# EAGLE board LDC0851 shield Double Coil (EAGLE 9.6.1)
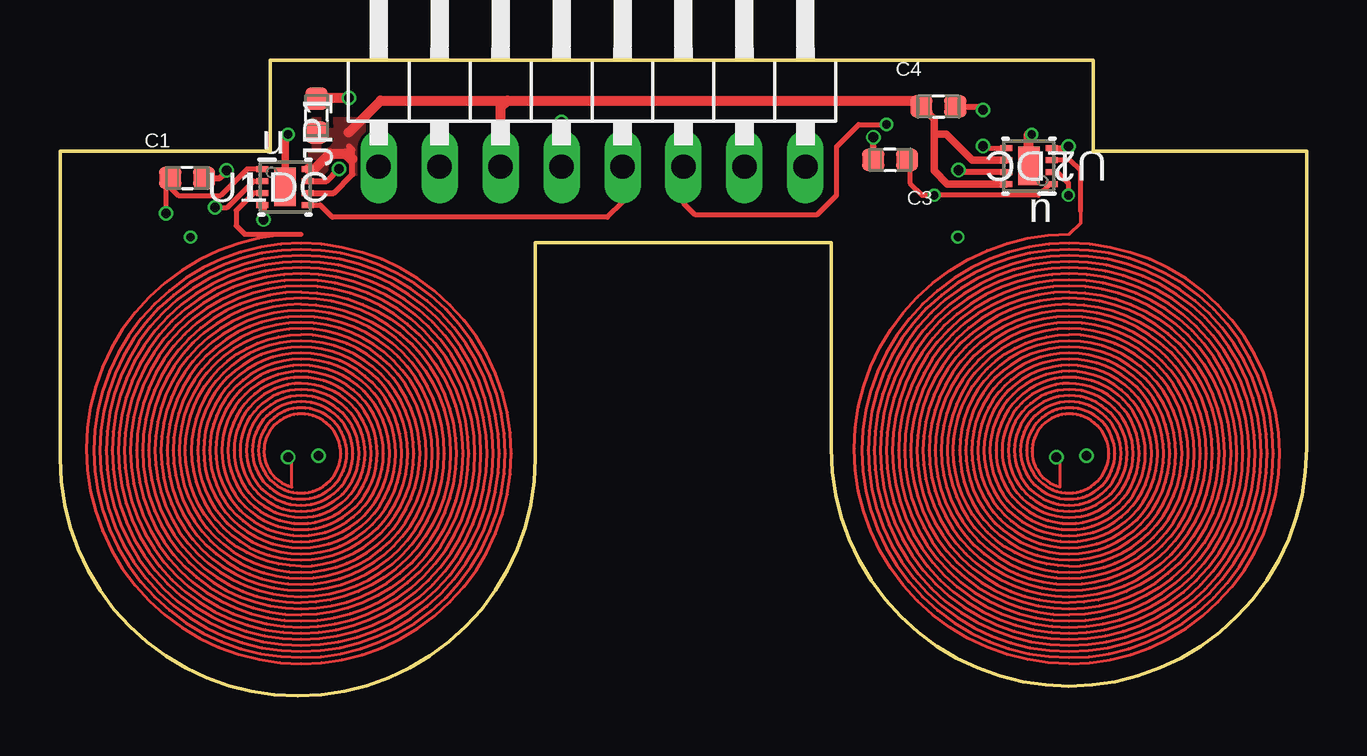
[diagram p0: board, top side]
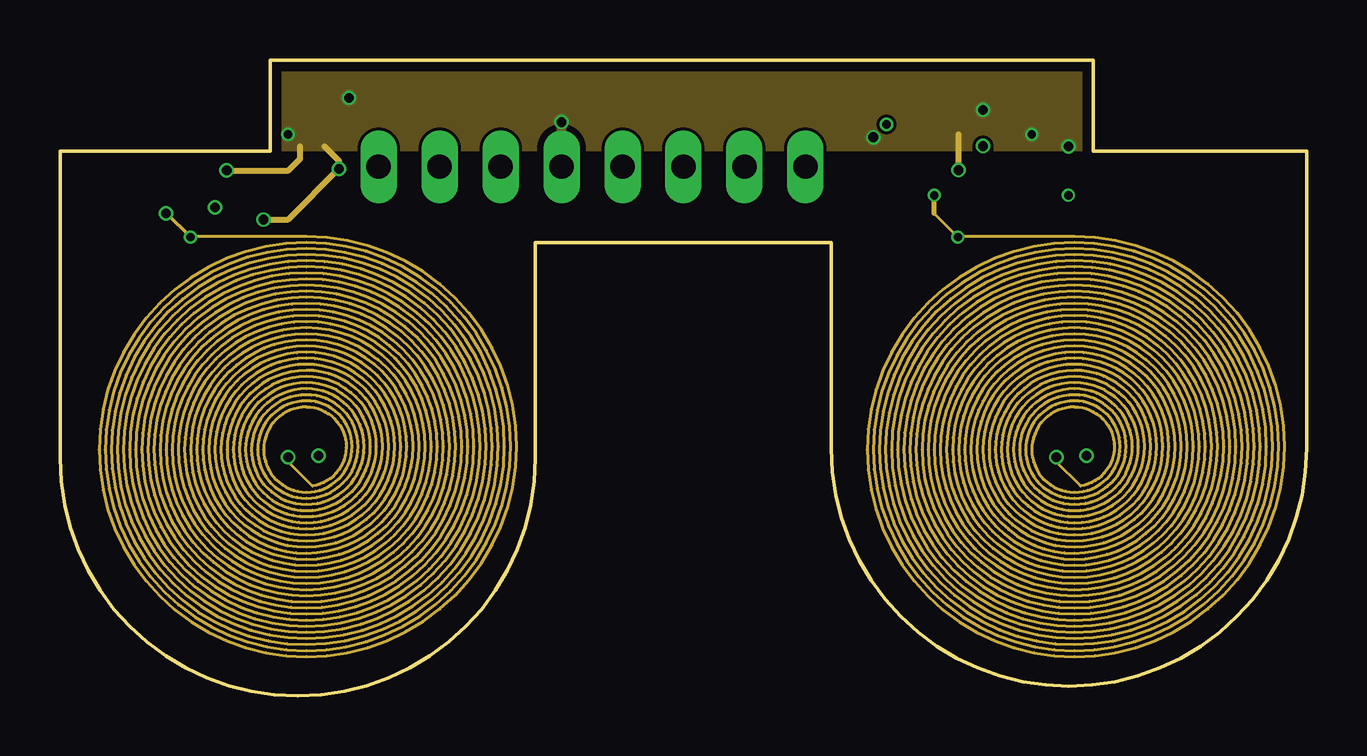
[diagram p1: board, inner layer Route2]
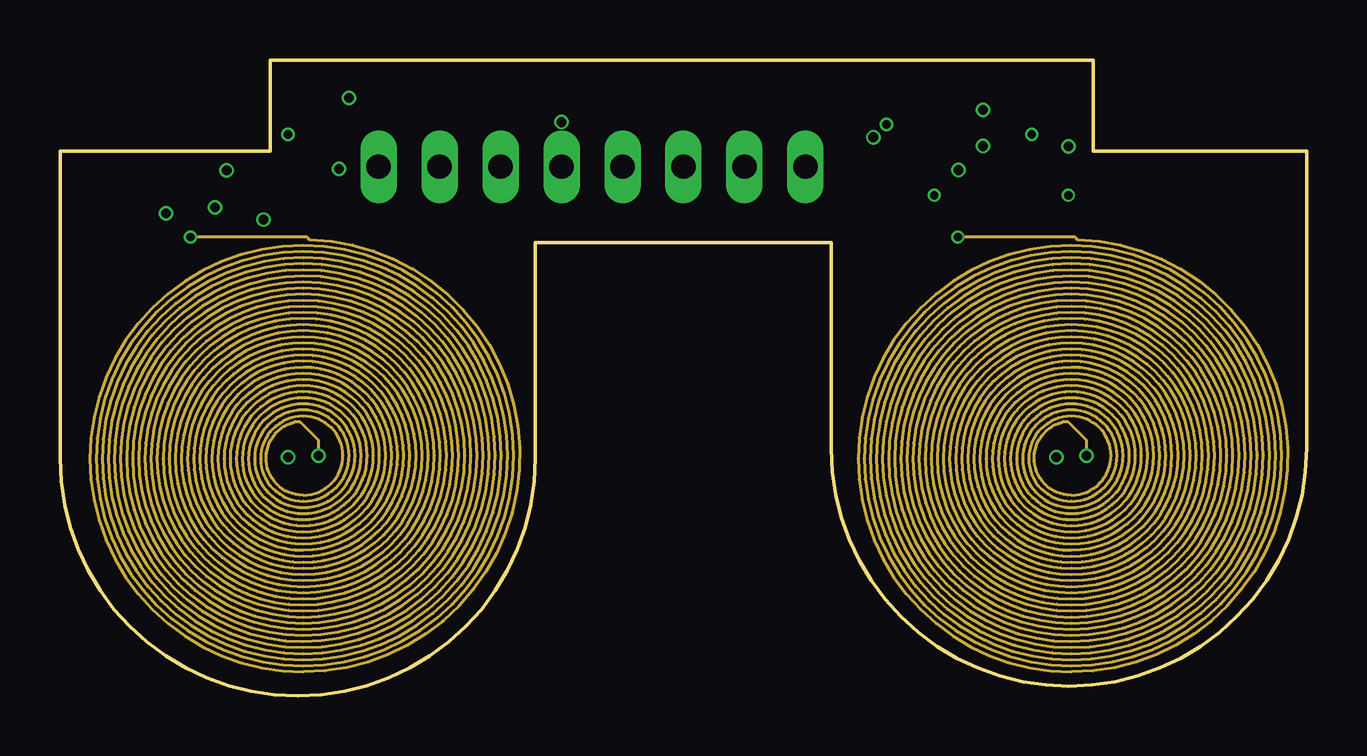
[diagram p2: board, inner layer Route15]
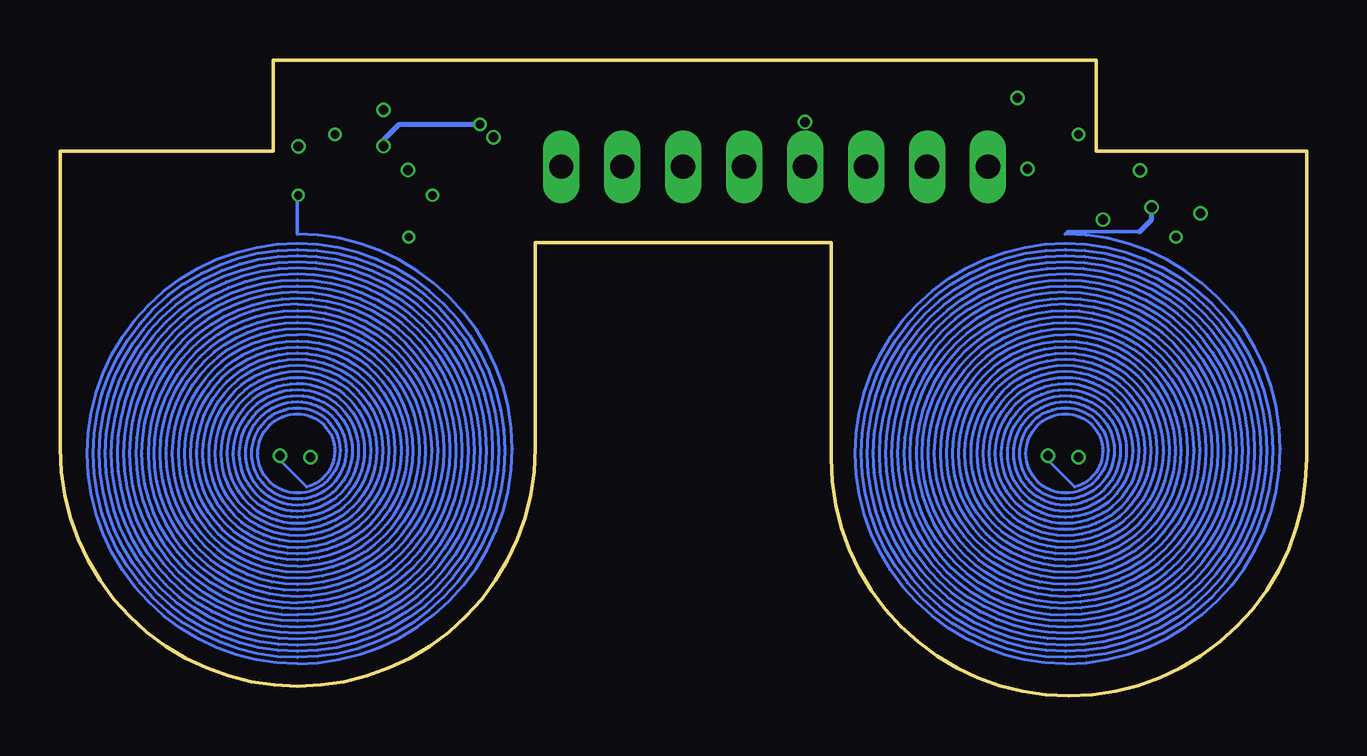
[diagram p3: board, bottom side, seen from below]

Size 51.94 x 26.52 mm. Coordinates in mm from the lower left corner, seen from the top.
Outline: 0,9.91 0,22.71 8.76,22.71 8.76,26.52 43.05,26.52 43.05,22.71 51.94,22.71 51.94,10.32 arc-180 32.13,10.32 32.13,18.9 19.81,18.9 19.81,9.91 arc-180 0,9.91
Copper layers (1*2*15*16): Top 0.035559375mm / dielectric 0.17018125mm / Route2 0.01778125mm / dielectric 47mil / Route15 0.01778125mm / dielectric 0.17018125mm / Bottom 0.035559375mm
Design rules "oshpark-4layer *": minimum track width 5mil, minimum drill 10mil, track to track 5mil, track to pad 5mil, pad to pad 5mil, via to via 5mil, smd to smd 5mil, copper to edge 15mil, drill to drill 6mil, minimum pad ring 4mil, minimum via ring 4mil, stop-mask expansion 2.5mil, vias tented up to drill 0mil, thermal gap 10mil

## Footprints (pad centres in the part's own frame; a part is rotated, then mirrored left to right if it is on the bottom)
CAP_0603 = smd 0.92 x 0.93: 1 -0.705,0; 2 0.705,0
1X08/90 = drill 1.016 long: 1 -8.89,-3.81; 2 -6.35,-3.81; 3 -3.81,-3.81; 4 -1.27,-3.81; 5 1.27,-3.81; 6 3.81,-3.81; 7 6.35,-3.81; 8 8.89,-3.81
DSG0008A = smd 0.5 x 0.25: 1 -0.95,0.75; 2 -0.95,0.25; 3 -0.95,-0.25; 4 -0.95,-0.75; 5 0.95,-0.75; 6 0.95,-0.25; 7 0.95,0.25; 8 0.95,0.75 | smd 0.9 x 1.6: 9 0,0 | smd 0.5 x 0.5: V 0,0.4

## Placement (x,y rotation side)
C1  68pF  [CAP_0603]  5.3,21.6 0 top
C2  .1uF  [CAP_0603]  10.69,24.2 90 top
C3  68pF  [CAP_0603]  34.59,22.35 180 top
C4  .1uF  [CAP_0603]  36.6,24.58 0 top
JP1  [1X08/90]  22.17,25.88 0 top
U1  LDC  [DSG0008A]  9.38,21.22 0 top
U2  LDC  [DSG0008A]  40.37,22.09 180 top

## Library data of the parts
C1-C4 = Resistor_Capacitor; CREATED_BY: PCBLayout.com; DIGIKEY_PART_NUMBER: 399-7814-2-ND; MANUFACTURER: KEMET; MPN: C0603C100C5GACTU; PACKAGE: SMD 0603
JP1 = pinhead
U1 U2 = LDC0851; ALTERNATE_PARTNUMBER: LDC0851DSGT; COMPTYPE: IC; MANUFACTURER: Texas Instruments; MOUNTTYPE: SMT; PACKAGEREFERENCE: DSG0008A; PARTNUMBER: LDC0851DSGR; PIN_COUNT: 9; REFDES: RefDes; TYPE: TYPE

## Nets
A0: JP1.5 U1.5
A1: JP1.6 U2.5
GND: C1.2 C2.2 C3.2 C4.2 JP1.4 U1.4 U1.7 U1.9 U2.4 U2.7 U2.9
L-COM: C1.1 U1.1 U1.2 U1.3
L-COM1: C3.1 U2.1 U2.2 U2.3
VDD: C2.1 C4.1 JP1.3 U1.6 U1.8 U2.6 U2.8

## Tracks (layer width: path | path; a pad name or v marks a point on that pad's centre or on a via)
A0
  Top 0.203: U1.5 10.84,20.47 11.34,19.96 22.81,19.96 23.44,20.59 JP1.5
A1  (via drill 0.35, 0.4 pad 0.6)
  Top 0.203: JP1.6 25.98,20.55 26.45,20.08 31.56,20.08 32.36,20.88 32.36,22.91 33.28,23.83 v34.44,23.83 | v38.46,22.92 38.54,22.84 U2.5
  Bottom 0.203: v34.44,23.83 37.82,23.83 38.46,23.19 v38.46,22.92
GND  (via drill 0.35, 0.4 pad 0.6)
  Top 0.254: C1.2 6.67,21.6 6.96,21.89 v6.95,21.91 | U1.7 11.11,21.47 v11.62,21.98 | U1.4 8.49,20.41 v8.49,19.86 | U2.4 41.95,22.84 v42.01,22.91 | U2.7 37.49,21.84 37.44,21.89 v37.44,21.92 | C3.2 33.88,22.91 33.89,22.91 v33.89,23.3 | C4.2 38.31,24.58 v38.46,24.43
  Top 0.305: U1.9 9.38,23.42 v9.5,23.42
  Top 0.406: C2.2 10.73,24.94 v12.04,24.94 | JP1.4 v20.9,23.93 | U2.9 40.37,23.42 v40.49,23.42
  Route2 0.254: v8.49,19.86 9.5,19.86 v11.62,21.98 11.62,22.31 11.03,22.91 | v6.95,21.91 9.52,21.91 10.01,22.4 10.01,22.91 | v37.44,21.92 37.44,23.42
  pour Route2: 8.49,26.47 43.03,26.47 43.03,22.91 8.49,22.91
L-COM  (via drill 0.35, 0.4 pad 0.51, 0.4 pad 0.6)
  Top 0.127: 10.05,19.25 arc180 10.05,1.35 arc180 10.05,18.87 arc180 10.05,1.6 arc180 10.05,18.62 arc180 10.05,1.86 arc180 10.05,18.37 arc180 10.05,2.11 arc180 10.05,18.11 arc180 10.05,2.36 arc180 10.05,17.86 arc180 10.05,2.62 arc180 10.05,17.6 arc180 10.05,2.87 arc180 10.05,17.35 arc180 10.05,3.13 arc180 10.05,17.1 arc180 10.05,3.38 arc180 10.05,16.84 arc180 10.05,3.63 arc180 10.05,16.59 arc180 10.05,3.89 arc180 10.05,16.33 arc180 10.05,4.14 arc180 10.05,16.08 arc180 10.05,4.4 arc180 10.05,15.83 arc180 10.05,4.65 arc180 10.05,15.57 arc180 10.05,4.9 arc180 10.05,15.32 arc180 10.05,5.16 arc180 10.05,15.06 arc180 10.05,5.41 arc180 10.05,14.81 arc180 10.05,5.67 arc180 10.05,14.56 arc180 10.05,5.92 arc180 10.05,14.3 arc180 10.05,6.17 arc180 10.05,14.05 arc180 10.05,6.43 arc180 10.05,13.79 arc180 10.05,6.68 arc180 10.05,13.54 arc180 10.05,6.94 arc180 10.05,13.29 arc180 10.05,7.19 arc180 10.05,13.03 arc180 10.05,7.44 arc180 10.05,12.78 arc180 10.05,7.7 arc180 10.05,12.52 arc180 10.05,7.95 arc180 10.05,12.27 arc180 10.05,8.21 arc180 10.05,12.02 arc180 10.05,8.46 arc180 10.05,11.76 arc166 9.67,8.71 9.67,9.95
  Top 0.203: U1.1 7.79,21.97 6.69,20.87 4.93,20.87 4.59,21.2 C1.1 4.59,21.59 4.63,21.55 4.42,21.34 v4.42,20.12 | 8.06,21.47 U1.2 | U1.3 8.07,20.97 7.34,20.24 7.34,19.61 7.7,19.25 10.05,19.25 | 9.67,9.95 v9.51,9.95 | v6.45,20.37 6.96,20.37 8.06,21.47 | 8.06,21.47
  Route2 0.127: 9.51,9.76 10.52,8.75 arc171 10.26,12.05 arc180 10.26,8.49 arc180 10.26,12.3 arc180 10.26,8.24 arc180 10.26,12.56 arc180 10.26,7.99 arc180 10.26,12.81 arc180 10.26,7.73 arc180 10.26,13.07 arc180 10.26,7.48 arc180 10.26,13.32 arc180 10.26,7.23 arc180 10.26,13.58 arc180 10.26,6.97 arc180 10.26,13.83 arc180 10.26,6.72 arc180 10.26,14.08 arc180 10.26,6.46 arc180 10.26,14.34 arc180 10.26,6.21 arc180 10.26,14.59 arc180 10.26,5.95 arc180 10.26,14.84 arc180 10.26,5.7 arc180 10.26,15.1 arc180 10.26,5.45 arc180 10.26,15.35 arc180 10.26,5.19 arc180 10.26,15.61 arc180 10.26,4.94 arc180 10.26,15.86 arc180 10.26,4.69 arc180 10.26,16.12 arc180 10.26,4.43 arc180 10.26,16.37 arc180 10.26,4.18 arc180 10.26,16.62 arc180 10.26,3.92 arc180 10.26,16.88 arc180 10.26,3.67 arc180 10.26,17.13 arc180 10.26,3.41 arc180 10.26,17.38 arc180 10.26,3.16 arc180 10.26,17.64 arc180 10.26,2.91 arc180 10.26,17.89 arc180 10.26,2.65 arc180 10.26,18.15 arc180 10.26,2.4 arc180 10.26,18.4 arc180 10.26,2.15 arc180 10.26,18.66 arc180 10.26,1.89 arc180 10.26,18.91 arc180 10.26,1.64 arc180 10.26,19.16 5.44,19.16
  Route2 0.152: 5.44,19.16 v5.44,19.13 4.45,20.12 v4.42,20.12
  Route2 0.203: 9.51,9.76 v9.51,9.95
  Route15 0.127: v10.77,10.02 10.77,10.65 10.01,11.42 9.76,11.42 arc166 10.14,8.37 arc180 10.14,11.67 arc180 10.14,8.11 arc180 10.14,11.92 arc180 10.14,7.86 arc180 10.14,12.18 arc180 10.14,7.61 arc180 10.14,12.43 arc180 10.14,7.35 arc180 10.14,12.69 arc180 10.14,7.1 arc180 10.14,12.94 arc180 10.14,6.84 arc180 10.14,13.19 arc180 10.14,6.59 arc180 10.14,13.45 arc180 10.14,6.34 arc180 10.14,13.7 arc180 10.14,6.08 arc180 10.14,13.96 arc180 10.14,5.83 arc180 10.14,14.21 arc180 10.14,5.57 arc180 10.14,14.46 arc180 10.14,5.32 arc180 10.14,14.72 arc180 10.14,5.07 arc180 10.14,14.97 arc180 10.14,4.81 arc180 10.14,15.23 arc180 10.14,4.56 arc180 10.14,15.48 arc180 10.14,4.3 arc180 10.14,15.73 arc180 10.14,4.05 arc180 10.14,15.99 arc180 10.14,3.8 arc180 10.14,16.24 arc180 10.14,3.54 arc180 10.14,16.5 arc180 10.14,3.29 arc180 10.14,16.75 arc180 10.14,3.03 arc180 10.14,17 arc180 10.14,2.78 arc180 10.14,17.26 arc180 10.14,2.53 arc180 10.14,17.51 arc180 10.14,2.27 arc180 10.14,17.77 arc180 10.14,2.02 arc180 10.14,18.02 arc180 10.14,1.76 arc180 10.14,18.27 arc180 10.14,1.51 arc180 10.14,18.53 arc180 10.14,1.26 arc180 10.14,18.78 arc180 10.14,1 arc178 10.39,19.04 10.3,19.13 v5.44,19.13 5.41,19.13
  Bottom 0.127: 10.05,19.25 arc180 10.05,1.35 arc180 10.05,18.87 arc180 10.05,1.6 arc180 10.05,18.62 arc180 10.05,1.86 arc180 10.05,18.37 arc180 10.05,2.11 arc180 10.05,18.11 arc180 10.05,2.36 arc180 10.05,17.86 arc180 10.05,2.62 arc180 10.05,17.6 arc180 10.05,2.87 arc180 10.05,17.35 arc180 10.05,3.13 arc180 10.05,17.1 arc180 10.05,3.38 arc180 10.05,16.84 arc180 10.05,3.63 arc180 10.05,16.59 arc180 10.05,3.89 arc180 10.05,16.33 arc180 10.05,4.14 arc180 10.05,16.08 arc180 10.05,4.4 arc180 10.05,15.83 arc180 10.05,4.65 arc180 10.05,15.57 arc180 10.05,4.9 arc180 10.05,15.32 arc180 10.05,5.16 arc180 10.05,15.06 arc180 10.05,5.41 arc180 10.05,14.81 arc180 10.05,5.67 arc180 10.05,14.56 arc180 10.05,5.92 arc180 10.05,14.3 arc180 10.05,6.17 arc180 10.05,14.05 arc180 10.05,6.43 arc180 10.05,13.79 arc180 10.05,6.68 arc180 10.05,13.54 arc180 10.05,6.94 arc180 10.05,13.29 arc180 10.05,7.19 arc180 10.05,13.03 arc180 10.05,7.44 arc180 10.05,12.78 arc180 10.05,7.7 arc180 10.05,12.52 arc180 10.05,7.95 arc180 10.05,12.27 arc180 10.05,8.21 arc180 10.05,12.02 arc180 10.05,8.46 arc180 10.05,11.76 arc166 9.67,8.71 10.77,9.82 v10.77,10.02
  Bottom 0.152: 10.05,19.25 9.95,19.35 6.96,19.35
  Bottom 0.203: 6.96,19.35 6.45,19.86 v6.45,20.37
L-COM1  (via drill 0.35, 0.4 pad 0.51, 0.4 pad 0.6)
  Top 0.127: 42.05,19.25 arc180 42.05,1.35 arc180 42.05,18.87 arc180 42.05,1.6 arc180 42.05,18.62 arc180 42.05,1.86 arc180 42.05,18.37 arc180 42.05,2.11 arc180 42.05,18.11 arc180 42.05,2.36 arc180 42.05,17.86 arc180 42.05,2.62 arc180 42.05,17.6 arc180 42.05,2.87 arc180 42.05,17.35 arc180 42.05,3.13 arc180 42.05,17.1 arc180 42.05,3.38 arc180 42.05,16.84 arc180 42.05,3.63 arc180 42.05,16.59 arc180 42.05,3.89 arc180 42.05,16.33 arc180 42.05,4.14 arc180 42.05,16.08 arc180 42.05,4.4 arc180 42.05,15.83 arc180 42.05,4.65 arc180 42.05,15.57 arc180 42.05,4.9 arc180 42.05,15.32 arc180 42.05,5.16 arc180 42.05,15.06 arc180 42.05,5.41 arc180 42.05,14.81 arc180 42.05,5.67 arc180 42.05,14.56 arc180 42.05,5.92 arc180 42.05,14.3 arc180 42.05,6.17 arc180 42.05,14.05 arc180 42.05,6.43 arc180 42.05,13.79 arc180 42.05,6.68 arc180 42.05,13.54 arc180 42.05,6.94 arc180 42.05,13.29 arc180 42.05,7.19 arc180 42.05,13.03 arc180 42.05,7.44 arc180 42.05,12.78 arc180 42.05,7.7 arc180 42.05,12.52 arc180 42.05,7.95 arc180 42.05,12.27 arc180 42.05,8.21 arc180 42.05,12.02 arc180 42.05,8.46 arc180 42.05,11.76 arc166 41.67,8.71 41.67,9.95
  Top 0.152: 42.05,19.25 42.52,19.72 42.52,20.23
  Top 0.203: 41.23,21.34 40.77,20.88 v36.43,20.88 35.92,20.88 35.41,21.39 35.41,22.24 C3.1 | v42.01,20.88 42.01,21.39 41.56,21.84 U2.2 | 42.52,20.23 42.52,21.9 42.08,22.34 U2.3 | 41.67,9.95 v41.51,9.95
  Top 0.254: 41.23,21.34 U2.1
  Route2 0.127: 41.51,9.76 42.52,8.75 arc171 42.27,12.05 arc180 42.27,8.49 arc180 42.27,12.3 arc180 42.27,8.24 arc180 42.27,12.56 arc180 42.27,7.99 arc180 42.27,12.81 arc180 42.27,7.73 arc180 42.27,13.07 arc180 42.27,7.48 arc180 42.27,13.32 arc180 42.27,7.23 arc180 42.27,13.58 arc180 42.27,6.97 arc180 42.27,13.83 arc180 42.27,6.72 arc180 42.27,14.08 arc180 42.27,6.46 arc180 42.27,14.34 arc180 42.27,6.21 arc180 42.27,14.59 arc180 42.27,5.95 arc180 42.27,14.84 arc180 42.27,5.7 arc180 42.27,15.1 arc180 42.27,5.45 arc180 42.27,15.35 arc180 42.27,5.19 arc180 42.27,15.61 arc180 42.27,4.94 arc180 42.27,15.86 arc180 42.27,4.69 arc180 42.27,16.12 arc180 42.27,4.43 arc180 42.27,16.37 arc180 42.27,4.18 arc180 42.27,16.62 arc180 42.27,3.92 arc180 42.27,16.88 arc180 42.27,3.67 arc180 42.27,17.13 arc180 42.27,3.41 arc180 42.27,17.38 arc180 42.27,3.16 arc180 42.27,17.64 arc180 42.27,2.91 arc180 42.27,17.89 arc180 42.27,2.65 arc180 42.27,18.15 arc180 42.27,2.4 arc180 42.27,18.4 arc180 42.27,2.15 arc180 42.27,18.66 arc180 42.27,1.89 arc180 42.27,18.91 arc180 42.27,1.64 arc180 42.27,19.16 37.44,19.16 v37.41,19.13 36.43,20.12
  Route2 0.203: 41.51,9.76 v41.51,9.95 | 36.43,20.12 v36.43,20.88
  Route15 0.127: v42.78,10.02 42.78,10.65 42.01,11.42 41.76,11.42 arc166 42.14,8.37 arc180 42.14,11.67 arc180 42.14,8.11 arc180 42.14,11.92 arc180 42.14,7.86 arc180 42.14,12.18 arc180 42.14,7.61 arc180 42.14,12.43 arc180 42.14,7.35 arc180 42.14,12.69 arc180 42.14,7.1 arc180 42.14,12.94 arc180 42.14,6.84 arc180 42.14,13.19 arc180 42.14,6.59 arc180 42.14,13.45 arc180 42.14,6.34 arc180 42.14,13.7 arc180 42.14,6.08 arc180 42.14,13.96 arc180 42.14,5.83 arc180 42.14,14.21 arc180 42.14,5.57 arc180 42.14,14.46 arc180 42.14,5.32 arc180 42.14,14.72 arc180 42.14,5.07 arc180 42.14,14.97 arc180 42.14,4.81 arc180 42.14,15.23 arc180 42.14,4.56 arc180 42.14,15.48 arc180 42.14,4.3 arc180 42.14,15.73 arc180 42.14,4.05 arc180 42.14,15.99 arc180 42.14,3.8 arc180 42.14,16.24 arc180 42.14,3.54 arc180 42.14,16.5 arc180 42.14,3.29 arc180 42.14,16.75 arc180 42.14,3.03 arc180 42.14,17 arc180 42.14,2.78 arc180 42.14,17.26 arc180 42.14,2.53 arc180 42.14,17.51 arc180 42.14,2.27 arc180 42.14,17.77 arc180 42.14,2.02 arc180 42.14,18.02 arc180 42.14,1.76 arc180 42.14,18.27 arc180 42.14,1.51 arc180 42.14,18.53 arc180 42.14,1.26 arc180 42.14,18.78 arc180 42.14,1 arc178 42.39,19.04 42.3,19.13 v37.41,19.13
  Bottom 0.127: 42.05,19.25 arc180 42.05,1.35 arc180 42.05,18.87 arc180 42.05,1.6 arc180 42.05,18.62 arc180 42.05,1.86 arc180 42.05,18.37 arc180 42.05,2.11 arc180 42.05,18.11 arc180 42.05,2.36 arc180 42.05,17.86 arc180 42.05,2.62 arc180 42.05,17.6 arc180 42.05,2.87 arc180 42.05,17.35 arc180 42.05,3.13 arc180 42.05,17.1 arc180 42.05,3.38 arc180 42.05,16.84 arc180 42.05,3.63 arc180 42.05,16.59 arc180 42.05,3.89 arc180 42.05,16.33 arc180 42.05,4.14 arc180 42.05,16.08 arc180 42.05,4.4 arc180 42.05,15.83 arc180 42.05,4.65 arc180 42.05,15.57 arc180 42.05,4.9 arc180 42.05,15.32 arc180 42.05,5.16 arc180 42.05,15.06 arc180 42.05,5.41 arc180 42.05,14.81 arc180 42.05,5.67 arc180 42.05,14.56 arc180 42.05,5.92 arc180 42.05,14.3 arc180 42.05,6.17 arc180 42.05,14.05 arc180 42.05,6.43 arc180 42.05,13.79 arc180 42.05,6.68 arc180 42.05,13.54 arc180 42.05,6.94 arc180 42.05,13.29 arc180 42.05,7.19 arc180 42.05,13.03 arc180 42.05,7.44 arc180 42.05,12.78 arc180 42.05,7.7 arc180 42.05,12.52 arc180 42.05,7.95 arc180 42.05,12.27 arc180 42.05,8.21 arc180 42.05,12.02 arc180 42.05,8.46 arc180 42.05,11.76 arc166 41.67,8.71 42.78,9.82 v42.78,10.02
  Bottom 0.152: 42.05,19.25 42.05,20.84 v42.01,20.88
VDD
  Top 0.254: 12.04,22.91 12.18,22.77 12.18,22.4 12.18,21.75 11.4,20.97 U1.6
  Top 0.305: U2.8 36.98,21.34 36.43,21.89 36.43,23.42 | 36.43,23.42 36.43,24.04 C4.1 | U2.6 38.01,22.34 36.93,23.42 36.43,23.42
  Top 0.406: 18.65,24.83 13.36,24.83 12.02,23.49 | 18.65,24.83 35.64,24.83 C4.1 | 18.65,24.83 18.36,24.54 JP1.3 | U1.8 10.59,21.97 11.24,22.62 11.89,22.62 12.1,22.4 12.18,22.4
  pour Top: 10.52,23.93 10.52,21.89 12.55,21.89 12.55,23.93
